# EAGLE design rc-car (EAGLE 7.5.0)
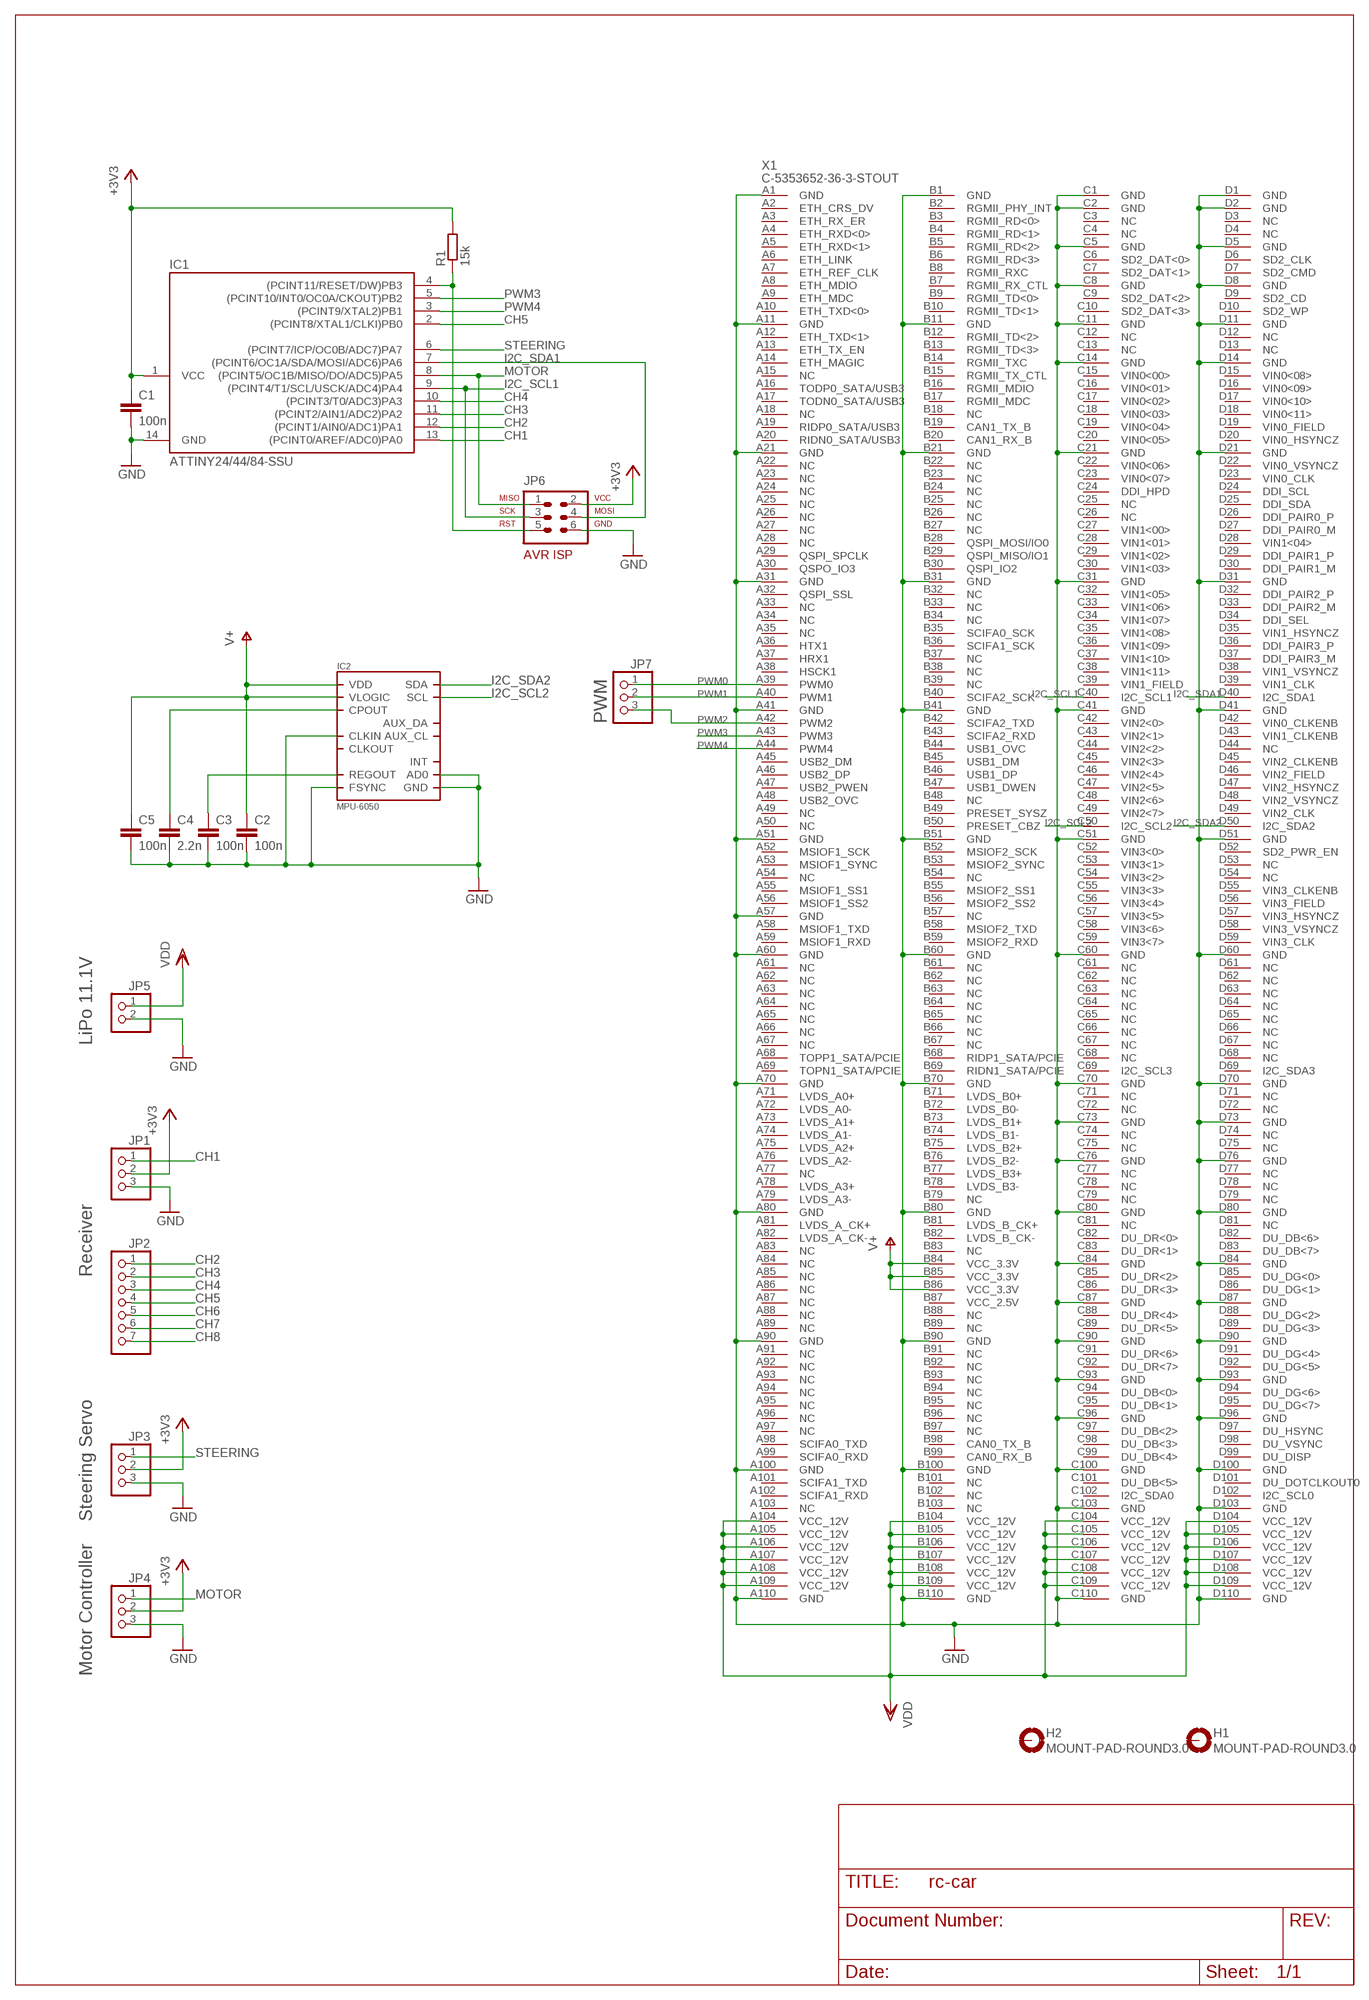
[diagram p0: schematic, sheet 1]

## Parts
C1  100n  C-EUC0805  [C0805]
C2  100n  C-EUC0805  [C0805]
C3  100n  C-EUC0805  [C0805]
C4  2.2n  C-EUC0805  [C0805]
C5  100n  C-EUC0805  [C0805]
H1  MOUNT-PAD-ROUND3.0  [3,0-PAD]
H2  MOUNT-PAD-ROUND3.0  [3,0-PAD]
IC1  ATTINY24/44/84-SSU  [SOIC14]
IC2  MPU-6050  [QFN.24.4X4]
JP1  PINHD-1X3/90  [1X03/90]
JP2  PINHD-1X7/90  [1X07/90]
JP3  PINHD-1X3/90  [1X03/90]
JP4  PINHD-1X3/90  [1X03/90]
JP5  PINHD-1X2  [1X02]
JP6  AVR-ISP-6HORZ  [AVR-ISP-6R]
JP7  PINHD-1X3  [1X03]
R1  15k  R-EU_M0805  [M0805]
X1  C-5353652-36-3-STOUT  [C-5353652-36-3]

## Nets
+3V3: C1.1 IC1.1(VCC) JP1.2 JP3.2 JP4.2 JP6.2 R1.2
CH1: IC1.13((PCINT0/AREF/ADC0)PA0) JP1.1
CH2: IC1.12((PCINT1/AIN0/ADC1)PA1) JP2.1
CH3: IC1.11((PCINT2/AIN1/ADC2)PA2) JP2.2
CH4: IC1.10((PCINT3/T0/ADC3)PA3) JP2.3
CH5: IC1.2((PCINT8/XTAL1/CLKI)PB0) JP2.4
CH6: JP2.5
CH7: JP2.6
CH8: JP2.7
GND: C1.2 C2.2 C3.2 C4.2 C5.2 IC1.14(GND) IC2.1(CLKIN) IC2.9(AD0) IC2.11(FSYNC) IC2.18(GND) JP1.3 JP3.3 JP4.3 JP5.2 JP6.6 X1.A1(GND) X1.A11(GND) X1.A21(GND) X1.A31(GND) X1.A41(GND) X1.A51(GND) X1.A57(GND) X1.A60(GND) X1.A70(GND) X1.A80(GND) X1.A90(GND) X1.A100(GND) X1.A110(GND) X1.B1(GND) X1.B11(GND) X1.B21(GND) X1.B31(GND) X1.B41(GND) X1.B51(GND) X1.B60(GND) X1.B70(GND) X1.B80(GND) X1.B90(GND) X1.B100(GND) X1.B110(GND) X1.C1(GND) X1.C2(GND) X1.C5(GND) X1.C8(GND) X1.C11(GND) X1.C14(GND) X1.C21(GND) X1.C31(GND) X1.C41(GND) X1.C51(GND) X1.C60(GND) X1.C70(GND) X1.C73(GND) X1.C76(GND) X1.C80(GND) X1.C84(GND) X1.C87(GND) X1.C90(GND) X1.C93(GND) X1.C96(GND) X1.C100(GND) X1.C103(GND) X1.C110(GND) X1.D1(GND) X1.D2(GND) X1.D5(GND) X1.D8(GND) X1.D11(GND) X1.D14(GND) X1.D21(GND) X1.D31(GND) X1.D41(GND) X1.D51(GND) X1.D60(GND) X1.D70(GND) X1.D73(GND) X1.D76(GND) X1.D80(GND) X1.D84(GND) X1.D87(GND) X1.D90(GND) X1.D93(GND) X1.D96(GND) X1.D100(GND) X1.D103(GND) X1.D110(GND)
I2C_SCL1: IC1.9((PCINT4/T1/SCL/USCK/ADC4)PA4) JP6.3 X1.C40(I2C_SCL1)
I2C_SCL2: IC2.23(SCL) X1.C50(I2C_SCL2)
I2C_SDA1: IC1.7((PCINT6/OC1A/SDA/MOSI/ADC6)PA6) JP6.4 X1.D40(I2C_SDA1)
I2C_SDA2: IC2.24(SDA) X1.D50(I2C_SDA2)
MOTOR: IC1.8((PCINT5/OC1B/MISO/DO/ADC5)PA5) JP4.1 JP6.1
N$2: IC1.4((PCINT11/RESET/DW)PB3) JP6.5 R1.1
N$4: C3.1 IC2.10(REGOUT)
N$5: C4.1 IC2.20(CPOUT)
PWM0: JP7.1 X1.A39(PWM0)
PWM1: JP7.2 X1.A40(PWM1)
PWM2: JP7.3 X1.A42(PWM2)
PWM3: IC1.5((PCINT10/INT0/OC0A/CKOUT)PB2) X1.A43(PWM3)
PWM4: IC1.3((PCINT9/XTAL2)PB1) X1.A44(PWM4)
STEERING: IC1.6((PCINT7/ICP/OC0B/ADC7)PA7) JP3.1
V+: C2.1 C5.1 IC2.8(VLOGIC) IC2.13(VDD) X1.B84(VCC_3.3V) X1.B85(VCC_3.3V) X1.B86(VCC_3.3V)
VDD: JP5.1 X1.A104(VCC_12V) X1.A105(VCC_12V) X1.A106(VCC_12V) X1.A107(VCC_12V) X1.A108(VCC_12V) X1.A109(VCC_12V) X1.B104(VCC_12V) X1.B105(VCC_12V) X1.B106(VCC_12V) X1.B107(VCC_12V) X1.B108(VCC_12V) X1.B109(VCC_12V) X1.C104(VCC_12V) X1.C105(VCC_12V) X1.C106(VCC_12V) X1.C107(VCC_12V) X1.C108(VCC_12V) X1.C109(VCC_12V) X1.D104(VCC_12V) X1.D105(VCC_12V) X1.D106(VCC_12V) X1.D107(VCC_12V) X1.D108(VCC_12V) X1.D109(VCC_12V)
Unconnected: H1.B3,0(MOUNT) H2.B3,0(MOUNT) IC2.6(AUX_DA) IC2.7(AUX_CL) IC2.12(INT) IC2.22(CLKOUT) X1.A2(ETH_CRS_DV) X1.A3(ETH_RX_ER) X1.A4(ETH_RXD<0>) X1.A5(ETH_RXD<1>) X1.A6(ETH_LINK) X1.A7(ETH_REF_CLK) X1.A8(ETH_MDIO) X1.A9(ETH_MDC) X1.A10(ETH_TXD<0>) X1.A12(ETH_TXD<1>) X1.A13(ETH_TX_EN) X1.A14(ETH_MAGIC) X1.A15(NC) X1.A16(TODP0_SATA/USB3) X1.A17(TODN0_SATA/USB3) X1.A18(NC) X1.A19(RIDP0_SATA/USB3) X1.A20(RIDN0_SATA/USB3) X1.A22(NC) X1.A23(NC) X1.A24(NC) X1.A25(NC) X1.A26(NC) X1.A27(NC) X1.A28(NC) X1.A29(QSPI_SPCLK) X1.A30(QSPO_IO3) X1.A32(QSPI_SSL) X1.A33(NC) X1.A34(NC) X1.A35(NC) X1.A36(HTX1) X1.A37(HRX1) X1.A38(HSCK1) X1.A45(USB2_DM) X1.A46(USB2_DP) X1.A47(USB2_PWEN) X1.A48(USB2_OVC) X1.A49(NC) X1.A50(NC) X1.A52(MSIOF1_SCK) X1.A53(MSIOF1_SYNC) X1.A54(NC) X1.A55(MSIOF1_SS1) X1.A56(MSIOF1_SS2) X1.A58(MSIOF1_TXD) X1.A59(MSIOF1_RXD) X1.A61(NC) X1.A62(NC) X1.A63(NC) X1.A64(NC) X1.A65(NC) X1.A66(NC) X1.A67(NC) X1.A68(TOPP1_SATA/PCIE) X1.A69(TOPN1_SATA/PCIE) X1.A71(LVDS_A0+) X1.A72(LVDS_A0-) X1.A73(LVDS_A1+) X1.A74(LVDS_A1-) X1.A75(LVDS_A2+) X1.A76(LVDS_A2-) X1.A77(NC) X1.A78(LVDS_A3+) X1.A79(LVDS_A3-) X1.A81(LVDS_A_CK+) X1.A82(LVDS_A_CK-) X1.A83(NC) X1.A84(NC) X1.A85(NC) X1.A86(NC) X1.A87(NC) X1.A88(NC) X1.A89(NC) X1.A91(NC) X1.A92(NC) X1.A93(NC) X1.A94(NC) X1.A95(NC) X1.A96(NC) X1.A97(NC) X1.A98(SCIFA0_TXD) X1.A99(SCIFA0_RXD) X1.A101(SCIFA1_TXD) X1.A102(SCIFA1_RXD) X1.A103(NC) X1.B2(RGMII_PHY_INT) X1.B3(RGMII_RD<0>) X1.B4(RGMII_RD<1>) X1.B5(RGMII_RD<2>) X1.B6(RGMII_RD<3>) X1.B7(RGMII_RX_CTL) X1.B8(RGMII_RXC) X1.B9(RGMII_TD<0>) X1.B10(RGMII_TD<1>) X1.B12(RGMII_TD<2>) X1.B13(RGMII_TD<3>) X1.B14(RGMII_TXC) X1.B15(RGMII_TX_CTL) X1.B16(RGMII_MDIO) X1.B17(RGMII_MDC) X1.B18(NC) X1.B19(CAN1_TX_B) X1.B20(CAN1_RX_B) X1.B22(NC) X1.B23(NC) X1.B24(NC) X1.B25(NC) X1.B26(NC) X1.B27(NC) X1.B28(QSPI_MOSI/IO0) X1.B29(QSPI_MISO/IO1) X1.B30(QSPI_IO2) X1.B32(NC) X1.B33(NC) X1.B34(NC) X1.B35(SCIFA0_SCK) X1.B36(SCIFA1_SCK) X1.B37(NC) X1.B38(NC) X1.B39(NC) X1.B40(SCIFA2_SCK) X1.B42(SCIFA2_TXD) X1.B43(SCIFA2_RXD) X1.B44(USB1_OVC) X1.B45(USB1_DM) X1.B46(USB1_DP) X1.B47(USB1_DWEN) X1.B48(NC) X1.B49(PRESET_SYSZ) X1.B50(PRESET_CBZ) X1.B52(MSIOF2_SCK) X1.B53(MSIOF2_SYNC) X1.B54(NC) X1.B55(MSIOF2_SS1) X1.B56(MSIOF2_SS2) X1.B57(NC) X1.B58(MSIOF2_TXD) X1.B59(MSIOF2_RXD) X1.B61(NC) X1.B62(NC) X1.B63(NC) X1.B64(NC) X1.B65(NC) X1.B66(NC) X1.B67(NC) X1.B68(RIDP1_SATA/PCIE) X1.B69(RIDN1_SATA/PCIE) X1.B71(LVDS_B0+) X1.B72(LVDS_B0-) X1.B73(LVDS_B1+) X1.B74(LVDS_B1-) X1.B75(LVDS_B2+) X1.B76(LVDS_B2-) X1.B77(LVDS_B3+) X1.B78(LVDS_B3-) X1.B79(NC) X1.B81(LVDS_B_CK+) X1.B82(LVDS_B_CK-) X1.B83(NC) X1.B87(VCC_2.5V) X1.B88(NC) X1.B89(NC) X1.B91(NC) X1.B92(NC) X1.B93(NC) X1.B94(NC) X1.B95(NC) X1.B96(NC) X1.B97(NC) X1.B98(CAN0_TX_B) X1.B99(CAN0_RX_B) X1.B101(NC) X1.B102(NC) X1.B103(NC) X1.C3(NC) X1.C4(NC) X1.C6(SD2_DAT<0>) X1.C7(SD2_DAT<1>) X1.C9(SD2_DAT<2>) X1.C10(SD2_DAT<3>) X1.C12(NC) X1.C13(NC) X1.C15(VIN0<00>) X1.C16(VIN0<01>) X1.C17(VIN0<02>) X1.C18(VIN0<03>) X1.C19(VIN0<04>) X1.C20(VIN0<05>) X1.C22(VIN0<06>) X1.C23(VIN0<07>) X1.C24(DDI_HPD) X1.C25(NC) X1.C26(NC) X1.C27(VIN1<00>) X1.C28(VIN1<01>) X1.C29(VIN1<02>) X1.C30(VIN1<03>) X1.C32(VIN1<05>) X1.C33(VIN1<06>) X1.C34(VIN1<07>) X1.C35(VIN1<08>) X1.C36(VIN1<09>) X1.C37(VIN1<10>) X1.C38(VIN1<11>) X1.C39(VIN1_FIELD) X1.C42(VIN2<0>) X1.C43(VIN2<1>) X1.C44(VIN2<2>) X1.C45(VIN2<3>) X1.C46(VIN2<4>) X1.C47(VIN2<5>) X1.C48(VIN2<6>) X1.C49(VIN2<7>) X1.C52(VIN3<0>) X1.C53(VIN3<1>) X1.C54(VIN3<2>) X1.C55(VIN3<3>) X1.C56(VIN3<4>) X1.C57(VIN3<5>) X1.C58(VIN3<6>) X1.C59(VIN3<7>) X1.C61(NC) X1.C62(NC) X1.C63(NC) X1.C64(NC) X1.C65(NC) X1.C66(NC) X1.C67(NC) X1.C68(NC) X1.C69(I2C_SCL3) X1.C71(NC) X1.C72(NC) X1.C74(NC) X1.C75(NC) X1.C77(NC) X1.C78(NC) X1.C79(NC) X1.C81(NC) X1.C82(DU_DR<0>) X1.C83(DU_DR<1>) X1.C85(DU_DR<2>) X1.C86(DU_DR<3>) X1.C88(DU_DR<4>) X1.C89(DU_DR<5>) X1.C91(DU_DR<6>) X1.C92(DU_DR<7>) X1.C94(DU_DB<0>) X1.C95(DU_DB<1>) X1.C97(DU_DB<2>) X1.C98(DU_DB<3>) X1.C99(DU_DB<4>) X1.C101(DU_DB<5>) X1.C102(I2C_SDA0) X1.D3(NC) X1.D4(NC) X1.D6(SD2_CLK) X1.D7(SD2_CMD) X1.D9(SD2_CD) X1.D10(SD2_WP) X1.D12(NC) X1.D13(NC) X1.D15(VIN0<08>) X1.D16(VIN0<09>) X1.D17(VIN0<10>) X1.D18(VIN0<11>) X1.D19(VIN0_FIELD) X1.D20(VIN0_HSYNCZ) X1.D22(VIN0_VSYNCZ) X1.D23(VIN0_CLK) X1.D24(DDI_SCL) X1.D25(DDI_SDA) X1.D26(DDI_PAIR0_P) X1.D27(DDI_PAIR0_M) X1.D28(VIN1<04>) X1.D29(DDI_PAIR1_P) X1.D30(DDI_PAIR1_M) X1.D32(DDI_PAIR2_P) X1.D33(DDI_PAIR2_M) X1.D34(DDI_SEL) X1.D35(VIN1_HSYNCZ) X1.D36(DDI_PAIR3_P) X1.D37(DDI_PAIR3_M) X1.D38(VIN1_VSYNCZ) X1.D39(VIN1_CLK) X1.D42(VIN0_CLKENB) X1.D43(VIN1_CLKENB) X1.D44(NC) X1.D45(VIN2_CLKENB) X1.D46(VIN2_FIELD) X1.D47(VIN2_HSYNCZ) X1.D48(VIN2_VSYNCZ) X1.D49(VIN2_CLK) X1.D52(SD2_PWR_EN) X1.D53(NC) X1.D54(NC) X1.D55(VIN3_CLKENB) X1.D56(VIN3_FIELD) X1.D57(VIN3_HSYNCZ) X1.D58(VIN3_VSYNCZ) X1.D59(VIN3_CLK) X1.D61(NC) X1.D62(NC) X1.D63(NC) X1.D64(NC) X1.D65(NC) X1.D66(NC) X1.D67(NC) X1.D68(NC) X1.D69(I2C_SDA3) X1.D71(NC) X1.D72(NC) X1.D74(NC) X1.D75(NC) X1.D77(NC) X1.D78(NC) X1.D79(NC) X1.D81(NC) X1.D82(DU_DB<6>) X1.D83(DU_DB<7>) X1.D85(DU_DG<0>) X1.D86(DU_DG<1>) X1.D88(DU_DG<2>) X1.D89(DU_DG<3>) X1.D91(DU_DG<4>) X1.D92(DU_DG<5>) X1.D94(DU_DG<6>) X1.D95(DU_DG<7>) X1.D97(DU_HSYNC) X1.D98(DU_VSYNC) X1.D99(DU_DISP) X1.D101(DU_DOTCLKOUT0) X1.D102(I2C_SCL0)

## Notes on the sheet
- PWM
- LiPo 11.1V
- Receiver
- Steering Servo
- Motor Controller

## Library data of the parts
C1-C5 = rcl:C-EU: CAPACITOR, European symbol
H1 H2 = holes:MOUNT-PAD-ROUND: MOUNTING PAD, round
IC1 = attiny24_44_84:ATTINY24/44/84
IC2 = MPU6050:MPU-6050
JP1 JP3 JP4 JP7 = pinhead:PINHD-1X3: PIN HEADER
JP2 = pinhead:PINHD-1X7: PIN HEADER
JP5 = pinhead:PINHD-1X2: PIN HEADER
JP6 = avr-7:AVR-ISP-6: AVR ISP-6 Serial Programming Header
R1 = rcl:R-EU_: RESISTOR, European symbol
X1 = con-tyco:C-5353652-36-3-STOUT

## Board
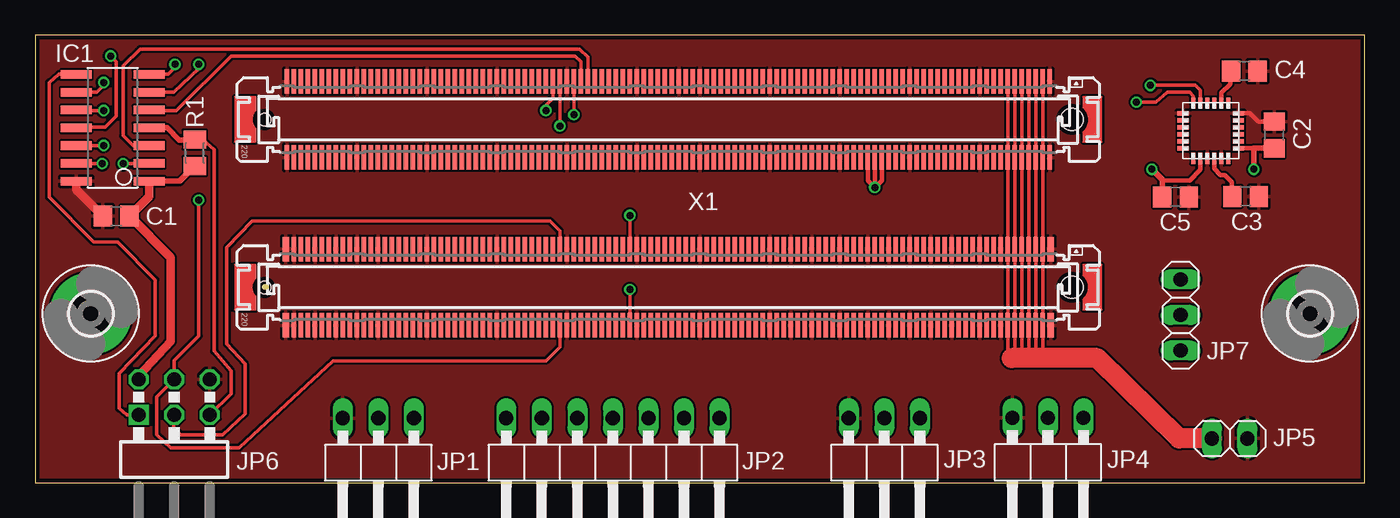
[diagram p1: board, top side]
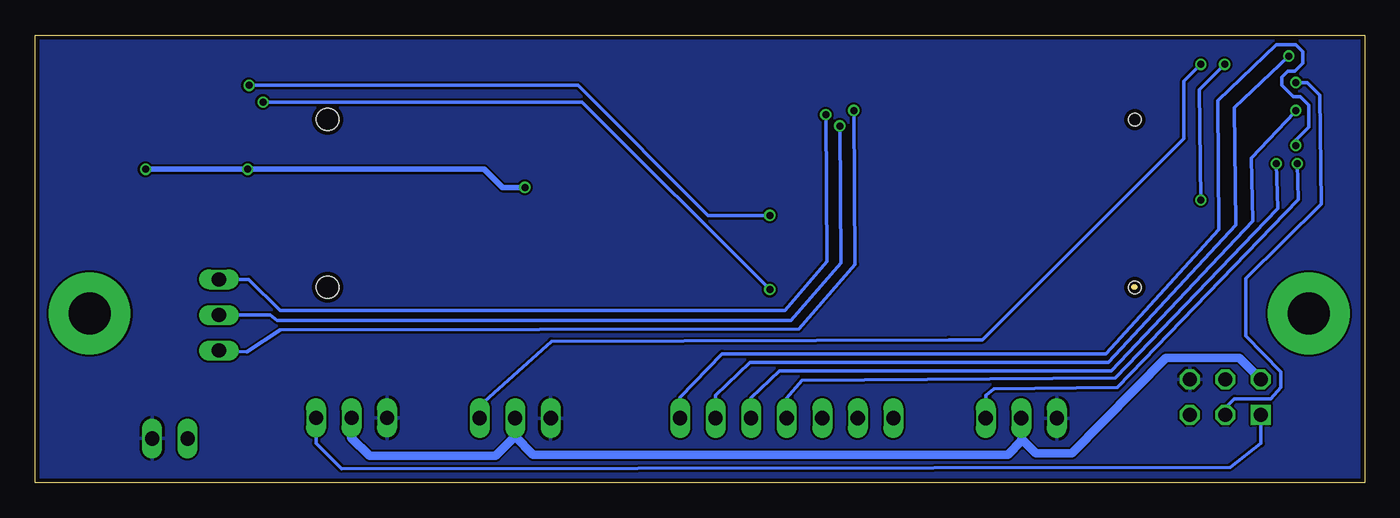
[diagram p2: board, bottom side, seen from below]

Size 95 x 32 mm. Coordinates in mm from the lower left corner, seen from the top.
Outline: 16.4,14 16.5,14
Outline: 0,0 95,0 95,32 0,32 0,0
Copper layers (1*16): Top 0.035mm / dielectric 1.5mm / Bottom 0.035mm
Design rules "PCB-POOL Standard": minimum track width 0.15mm, minimum drill 0.3mm, track to track 0.15mm, track to pad 0.15mm, pad to pad 0.15mm, via to via 0.15mm, smd to smd 0.15mm, copper to edge 0.3mm, drill to drill 0.2mm, minimum pad ring 0.2mm, minimum via ring 0.15mm, stop-mask expansion 0.075mm, vias tented up to drill 0mil, thermal gap 0.2mm

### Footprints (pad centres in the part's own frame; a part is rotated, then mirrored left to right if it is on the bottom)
C0805 = smd 1.3 x 1.5: 1 -0.95,0; 2 0.95,0
3,0-PAD = drill 3 pad 5.842: B3,0 0,0
SOIC14 = smd 0.61 x 2.21: 1 -3.81,-2.603; 2 -2.54,-2.603; 3 -1.27,-2.603; 4 0,-2.603; 5 1.27,-2.603; 6 2.54,-2.603; 7 3.81,-2.603; 8 3.81,2.603; 9 2.54,2.603; 10 1.27,2.603; 11 0,2.603; 12 -1.27,2.603; 13 -2.54,2.603; 14 -3.81,2.603
QFN.24.4X4 = smd 0.8 x 0.3: 1 -1.975,1.25; 2 -1.975,0.75; 3 -1.975,0.25; 4 -1.975,-0.25; 5 -1.975,-0.75; 6 -1.975,-1.25; 13 1.975,-1.25; 14 1.975,-0.75; 15 1.975,-0.25; 16 1.975,0.25; 17 1.975,0.75; 18 1.975,1.25 | smd 0.3 x 0.8: 7 -1.25,-1.975; 8 -0.75,-1.975; 9 -0.25,-1.975; 10 0.25,-1.975; 11 0.75,-1.975; 12 1.25,-1.975; 19 1.25,1.975; 20 0.75,1.975; 21 0.25,1.975; 22 -0.25,1.975; 23 -0.75,1.975; 24 -1.25,1.975
1X03/90 = drill 1.016 long: 1 -2.54,-3.81; 2 0,-3.81; 3 2.54,-3.81
1X07/90 = drill 1.016 long: 1 -7.62,-3.81; 2 -5.08,-3.81; 3 -2.54,-3.81; 4 0,-3.81; 5 2.54,-3.81; 6 5.08,-3.81; 7 7.62,-3.81
1X02 = drill 1.016 long: 1 -1.27,0; 2 1.27,0
AVR-ISP-6R = drill 1.016 square: 1 -2.54,-1.27 | drill 1.016 octagon: 2 -2.54,1.27; 3 0,-1.27; 4 0,1.27; 5 2.54,-1.27; 6 2.54,1.27
1X03 = drill 1.016 long: 1 -2.54,0; 2 0,0; 3 2.54,0
M0805 = smd 1.3 x 1.6: 1 -0.95,0; 2 0.95,0
C-5353652-36-3 = smd 0.3 x 1.75: A1 -27.25,8.705; A2 -26.75,8.705; A3 -26.25,8.705; A4 -25.75,8.705; A5 -25.25,8.705; A6 -24.75,8.705; A7 -24.25,8.705; A8 -23.75,8.705; A9 -23.25,8.705; A10 -22.75,8.705; A11 -22.25,8.705; A12 -21.75,8.705; A13 -21.25,8.705; A14 -20.75,8.705; A15 -20.25,8.705; A16 -19.75,8.705; A17 -19.25,8.705; A18 -18.75,8.705; A19 -18.25,8.705; A20 -17.75,8.705; A21 -17.25,8.705; A22 -16.75,8.705; A23 -16.25,8.705; A24 -15.75,8.705; A25 -15.25,8.705; A26 -14.75,8.705; A27 -14.25,8.705; A28 -13.75,8.705; A29 -13.25,8.705; A30 -12.75,8.705; A31 -12.25,8.705; A32 -11.75,8.705; A33 -11.25,8.705; A34 -10.75,8.705; A35 -10.25,8.705; A36 -9.75,8.705; A37 -9.25,8.705; A38 -8.75,8.705; A39 -8.25,8.705; A40 -7.75,8.705; A41 -7.25,8.705; A42 -6.75,8.705; A43 -6.25,8.705; A44 -5.75,8.705; A45 -5.25,8.705; A46 -4.75,8.705; A47 -4.25,8.705; A48 -3.75,8.705; A49 -3.25,8.705; A50 -2.75,8.705; A51 -2.25,8.705; A52 -1.75,8.705; A53 -1.25,8.705; A54 -0.75,8.705; A55 -0.25,8.705; A56 0.25,8.705; A57 0.75,8.705; A58 1.25,8.705; A59 1.75,8.705; A60 2.25,8.705; A61 2.75,8.705; A62 3.25,8.705; A63 3.75,8.705; A64 4.25,8.705; A65 4.75,8.705; A66 5.25,8.705; A67 5.75,8.705; A68 6.25,8.705; A69 6.75,8.705; A70 7.25,8.705; A71 7.75,8.705; A72 8.25,8.705; A73 8.75,8.705; A74 9.25,8.705; A75 9.75,8.705; A76 10.25,8.705; A77 10.75,8.705; A78 11.25,8.705; A79 11.75,8.705; A80 12.25,8.705; A81 12.75,8.705; A82 13.25,8.705; A83 13.75,8.705; A84 14.25,8.705; A85 14.75,8.705; A86 15.25,8.705; A87 15.75,8.705; A88 16.25,8.705; A89 16.75,8.705; A90 17.25,8.705; A91 17.75,8.705; A92 18.25,8.705; A93 18.75,8.705; A94 19.25,8.705; A95 19.75,8.705; A96 20.25,8.705; A97 20.75,8.705; A98 21.25,8.705; A99 21.75,8.705; A100 22.25,8.705; A101 22.75,8.705; A102 23.25,8.705; A103 23.75,8.705; A104 24.25,8.705; A105 24.75,8.705; A106 25.25,8.705; A107 25.75,8.705; A108 26.25,8.705; A109 26.75,8.705; A110 27.25,8.705; B1 -27.25,3.275; B2 -26.75,3.275; B3 -26.25,3.275; B4 -25.75,3.275; B5 -25.25,3.275; B6 -24.75,3.275; B7 -24.25,3.275; B8 -23.75,3.275; B9 -23.25,3.275; B10 -22.75,3.275; B11 -22.25,3.275; B12 -21.75,3.275; B13 -21.25,3.275; B14 -20.75,3.275; B15 -20.25,3.275; B16 -19.75,3.275; B17 -19.25,3.275; B18 -18.75,3.275; B19 -18.25,3.275; B20 -17.75,3.275; B21 -17.25,3.275; B22 -16.75,3.275; B23 -16.25,3.275; B24 -15.75,3.275; B25 -15.25,3.275; B26 -14.75,3.275; B27 -14.25,3.275; B28 -13.75,3.275; B29 -13.25,3.275; B30 -12.75,3.275; B31 -12.25,3.275; B32 -11.75,3.275; B33 -11.25,3.275; B34 -10.75,3.275; B35 -10.25,3.275; B36 -9.75,3.275; B37 -9.25,3.275; B38 -8.75,3.275; B39 -8.25,3.275; B40 -7.75,3.275; B41 -7.25,3.275; B42 -6.75,3.275; B43 -6.25,3.275; B44 -5.75,3.275; B45 -5.25,3.275; B46 -4.75,3.275; B47 -4.25,3.275; B48 -3.75,3.275; B49 -3.25,3.275; B50 -2.75,3.275; B51 -2.25,3.275; B52 -1.75,3.275; B53 -1.25,3.275; B54 -0.75,3.275; B55 -0.25,3.275; B56 0.25,3.275; B57 0.75,3.275; B58 1.25,3.275; B59 1.75,3.275; B60 2.25,3.275; B61 2.75,3.275; B62 3.25,3.275; B63 3.75,3.275; B64 4.25,3.275; B65 4.75,3.275; B66 5.25,3.275; B67 5.75,3.275; B68 6.25,3.275; B69 6.75,3.275; B70 7.25,3.275; B71 7.75,3.275; B72 8.25,3.275; B73 8.75,3.275; B74 9.25,3.275; B75 9.75,3.275; B76 10.25,3.275; B77 10.75,3.275; B78 11.25,3.275; B79 11.75,3.275; B80 12.25,3.275; B81 12.75,3.275; B82 13.25,3.275; B83 13.75,3.275; B84 14.25,3.275; B85 14.75,3.275; B86 15.25,3.275; B87 15.75,3.275; B88 16.25,3.275; B89 16.75,3.275; B90 17.25,3.275; B91 17.75,3.275; B92 18.25,3.275; B93 18.75,3.275; B94 19.25,3.275; B95 19.75,3.275; B96 20.25,3.275; B97 20.75,3.275; B98 21.25,3.275; B99 21.75,3.275; B100 22.25,3.275; B101 22.75,3.275; B102 23.25,3.275; B103 23.75,3.275; B104 24.25,3.275; B105 24.75,3.275; B106 25.25,3.275; B107 25.75,3.275; B108 26.25,3.275; B109 26.75,3.275; B110 27.25,3.275; C2 -26.75,-3.275; C3 -26.25,-3.275; C4 -25.75,-3.275; C5 -25.25,-3.275; C6 -24.75,-3.275; C7 -24.25,-3.275; C8 -23.75,-3.275; C9 -23.25,-3.275; C10 -22.75,-3.275; C11 -22.25,-3.275; C12 -21.75,-3.275; C13 -21.25,-3.275; C14 -20.75,-3.275; C15 -20.25,-3.275; C16 -19.75,-3.275; C17 -19.25,-3.275; C18 -18.75,-3.275; C19 -18.25,-3.275; C20 -17.75,-3.275; C21 -17.25,-3.275; C22 -16.75,-3.275; C23 -16.25,-3.275; C24 -15.75,-3.275; C25 -15.25,-3.275; C26 -14.75,-3.275; C27 -14.25,-3.275; C28 -13.75,-3.275; C29 -13.25,-3.275; C30 -12.75,-3.275; C31 -12.25,-3.275; C32 -11.75,-3.275; C33 -11.25,-3.275; C34 -10.75,-3.275; C35 -10.25,-3.275; C36 -9.75,-3.275; C37 -9.25,-3.275; C38 -8.75,-3.275; C39 -8.25,-3.275; C40 -7.75,-3.275; C41 -7.25,-3.275; C42 -6.75,-3.275; C43 -6.25,-3.275; C44 -5.75,-3.275; C45 -5.25,-3.275; C46 -4.75,-3.275; C47 -4.25,-3.275; C48 -3.75,-3.275; C49 -3.25,-3.275; C50 -2.75,-3.275; C51 -2.25,-3.275; C52 -1.75,-3.275; C53 -1.25,-3.275; C54 -0.75,-3.275; C55 -0.25,-3.275; C56 0.25,-3.275; C57 0.75,-3.275; C58 1.25,-3.275; C59 1.75,-3.275; C60 2.25,-3.275; C61 2.75,-3.275; C62 3.25,-3.275; C63 3.75,-3.275; C64 4.25,-3.275; C65 4.75,-3.275; C66 5.25,-3.275; C67 5.75,-3.275; C68 6.25,-3.275; C69 6.75,-3.275; C70 7.25,-3.275; C71 7.75,-3.275; C72 8.25,-3.275; C73 8.75,-3.275; C74 9.25,-3.275; C75 9.75,-3.275; C76 10.25,-3.275; C77 10.75,-3.275; C78 11.25,-3.275; C79 11.75,-3.275; C80 12.25,-3.275; C81 12.75,-3.275; C82 13.25,-3.275; C83 13.75,-3.275; C84 14.25,-3.275; C85 14.75,-3.275; C86 15.25,-3.275; C87 15.75,-3.275; C88 16.25,-3.275; C89 16.75,-3.275; C90 17.25,-3.275; C91 17.75,-3.275; C92 18.25,-3.275; C93 18.75,-3.275; C94 19.25,-3.275; C95 19.75,-3.275; C96 20.25,-3.275; C97 20.75,-3.275; C98 21.25,-3.275; C99 21.75,-3.275; C100 22.25,-3.275; C101 22.75,-3.275; C102 23.25,-3.275; C103 23.75,-3.275; C104 24.25,-3.275; C105 24.75,-3.275; C106 25.25,-3.275; C107 25.75,-3.275; C108 26.25,-3.275; C109 26.75,-3.275; D2 -26.75,-8.725; D3 -26.25,-8.725; D4 -25.75,-8.725; D5 -25.25,-8.725; D6 -24.75,-8.725; D7 -24.25,-8.725; D8 -23.75,-8.725; D9 -23.25,-8.725; D10 -22.75,-8.725; D11 -22.25,-8.725; D12 -21.75,-8.725; D13 -21.25,-8.725; D14 -20.75,-8.725; D15 -20.25,-8.725; D16 -19.75,-8.725; D17 -19.25,-8.725; D18 -18.75,-8.725; D19 -18.25,-8.725; D20 -17.75,-8.725; D21 -17.25,-8.725; D22 -16.75,-8.725; D23 -16.25,-8.725; D24 -15.75,-8.725; D25 -15.25,-8.725; D26 -14.75,-8.725; D27 -14.25,-8.725; D28 -13.75,-8.725; D29 -13.25,-8.725; D30 -12.75,-8.725; D31 -12.25,-8.725; D32 -11.75,-8.725; D33 -11.25,-8.725; D34 -10.75,-8.725; D35 -10.25,-8.725; D36 -9.75,-8.725; D37 -9.25,-8.725; D38 -8.75,-8.725; D39 -8.25,-8.725; D40 -7.75,-8.725; D41 -7.25,-8.725; D42 -6.75,-8.725; D43 -6.25,-8.725; D44 -5.75,-8.725; D45 -5.25,-8.725; D46 -4.75,-8.725; D47 -4.25,-8.725; D48 -3.75,-8.725; D49 -3.25,-8.725; D50 -2.75,-8.725; D51 -2.25,-8.725; D52 -1.75,-8.725; D53 -1.25,-8.725; D54 -0.75,-8.725; D55 -0.25,-8.725; D56 0.25,-8.725; D57 0.75,-8.725; D58 1.25,-8.725; D59 1.75,-8.725; D60 2.25,-8.725; D61 2.75,-8.725; D62 3.25,-8.725; D63 3.75,-8.725; D64 4.25,-8.725; D65 4.75,-8.725; D66 5.25,-8.725; D67 5.75,-8.725; D68 6.25,-8.725; D69 6.75,-8.725; D70 7.25,-8.725; D71 7.75,-8.725; D72 8.25,-8.725; D73 8.75,-8.725; D74 9.25,-8.725; D75 9.75,-8.725; D76 10.25,-8.725; D77 10.75,-8.725; D78 11.25,-8.725; D79 11.75,-8.725; D80 12.25,-8.725; D81 12.75,-8.725; D82 13.25,-8.725; D83 13.75,-8.725; D84 14.25,-8.725; D85 14.75,-8.725; D86 15.25,-8.725; D87 15.75,-8.725; D88 16.25,-8.725; D89 16.75,-8.725; D90 17.25,-8.725; D91 17.75,-8.725; D92 18.25,-8.725; D93 18.75,-8.725; D94 19.25,-8.725; D95 19.75,-8.725; D96 20.25,-8.725; D97 20.75,-8.725; D98 21.25,-8.725; D99 21.75,-8.725; D100 22.25,-8.725; D101 22.75,-8.725; D102 23.25,-8.725; D103 23.75,-8.725; D104 24.25,-8.725; D105 24.75,-8.725; D106 25.25,-8.725; D107 25.75,-8.725; D108 26.25,-8.725; D109 26.75,-8.725 | smd 0.45 x 1.75: C1 -27.325,-3.275; C110 27.325,-3.275; D1 -27.325,-8.725; D110 27.325,-8.725 | hole 0.9: -28.85,-6; -28.85,6; -28.85,-6 | hole 1.6: 28.85,-6; 28.85,6; 28.85,-6

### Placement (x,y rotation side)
C1  5.8,19.05 180 top
C2  88.55,24.85 90 top
C3  86.5,20.45 0 top
C4  86.41,29.42 0 top
C5  81.49,20.42 0 top
H1  3.99,12.08 0 top
H2  91.1,12.08 0 top
IC1  5.55,25.36 90 top
IC2  84.01,25.15 0 top
JP1  24.53,0.79 180 top
JP2  41.29,0.79 180 top
JP3  60.69,0.79 180 top
JP4  72.38,0.81 180 top
JP5  85.36,3.15 0 top
JP6  9.95,6.1 0 top
JP7  81.85,11.98 90 top
R1  11.42,23.57 270 top
X1  45.25,19.96 0 top

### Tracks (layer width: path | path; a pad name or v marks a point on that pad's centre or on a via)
+3V3
  Top 0.406: IC1.1 10.35,21.55 R1.2
  Top 0.61: IC1.1 8.15,20.45 C1.1 9.7,16.1 9.7,10.1 7.41,7.61 JP6.2
  Bottom 0.61: JP4.2 72.4,4.6 72.4,3.2 71.1,1.9 62.1,1.9 60.69,3.31 JP3.2 60.7,3.3 59.4,2 25.5,2 24.53,2.97 JP1.2 24.5,4.57 24.5,3.1 23.5,2.1 20.9,2.1 14.2,8.9 8.94,8.9 JP6.2 7.41,7.39 7.4,7.4
CH1  (via drill 0.5)
  Top 0.254: v4.8,22.8 2.93,22.8 IC1.13
  Bottom 0.254: JP1.1 27.07,6.23 26.5,6.7 17.67,6.8 4.75,20.22 4.82,22.82 v4.8,22.8
CH2  (via drill 0.5)
  Top 0.254: IC1.12 2.94,24.1 v4.9,24.1
  Bottom 0.254: JP2.1 48.91,6.09 45.9,9.2 18.5,9.2 10.4,18.1 10.5,27.3 6.3,31.3 4.9,31.3 4.4,30.8 4.4,30 5,29.4 5.5,29.4 5.9,29 5.9,28.4 5.1,27.6 4.6,27.6 4,27 4,25.4 4.9,24.5 v4.9,24.1
CH3  (via drill 0.5)
  Top 0.254: IC1.11 2.99,25.4 5,25.4 5.8,26.2 5.8,30.1 v5.4,30.5
  Bottom 0.254: JP2.2 46.37,6.23 43.9,8.6 18.3,8.6 9.2,18.4 9.3,26.8 v5.4,30.5
CH4  (via drill 0.5)
  Top 0.254: v4.9,26.6 2.88,26.6 IC1.10
  Bottom 0.254: JP2.3 43.83,6.07 41.8,8 18.1,8 8,18.7 8.1,23.2 5,26.5 | 5,26.5 5.1,26.5 | 5,26.5 v4.9,26.6
CH5  (via drill 0.5)
  Top 0.254: v6.3,22.8 8.13,22.8 IC1.2
  Bottom 0.254: JP2.4 41.29,6.01 40.2,7.3 17.8,7.5 6.2,19.6 v6.3,22.8
GND
  Top 0.305: IC2.18 86.8,26.4 87.4,25.8 C2.2
  Top 0.61: IC1.14 2.95,20.95 C1.2
  pour Top: 0.2,31.8 94.8,31.8 94.8,0.2 0.2,0.2 0.2,31.7
  pour Bottom: 0.3,31.7 94.7,31.7 94.7,0.4 0.3,0.4 0.3,31.6
I2C_SCL1  (via drill 0.5)
  Top 0.254: X1.C40 37.5,18 36.8,18.7 15.5,18.7 13.7,16.8 13.7,9.9 15,8.5 15,4.9 13.4,3.4 10.4,3.4 9.9,3.9 9.9,4.78 JP6.3 | v4.9,28.6 4.9,28.4 4.4,27.9 IC1.9
  Bottom 0.254: JP6.3 9.95,5.35 9.3,6 6.7,6 6,6.8 6,7.9 8.5,10.5 8.5,14.6 3.1,19.9 3.2,27.7 4.1,28.6 v4.9,28.6
I2C_SCL2  (via drill 0.5)
  Top 0.254: IC2.23 83.26,28.04 82.9,28.4 v79.7,28.4 | v42.5,19.1 X1.C50
  Bottom 0.254: v79.7,28.4 56.2,28.4 46.9,19.1 v42.5,19.1
I2C_SDA1  (via drill 0.5)
  Top 0.254: X1.D40 37.5,9.7 36.5,8.7 21.3,8.7 14.6,2.5 9.7,2.5 8.7,3.4 8.7,6.12 JP6.4 9.95,8.75 11.7,10.5 v11.7,20.2 | v10,29.9 9.9,29.6 9.5,29.2 8.18,29.2 IC1.7
  Bottom 0.254: v11.7,20.2 11.8,28.1 v10,29.9
I2C_SDA2  (via drill 0.5)
  Top 0.254: IC2.24 82.78,27.62 82.5,27.9 80.9,27.9 80.1,27.2 v78.7,27.2 | v42.5,13.8 X1.D50
  Bottom 0.254: v78.7,27.2 55.9,27.2 v42.5,13.8
MOTOR
  Top 0.254: JP6.1 6.57,4.83 6,5.3 6,7.8 8.6,10.5 8.6,14.5 5.9,17.2 4.2,17.2 1,20.4 1,28.6 1.7,29.2 2.92,29.2 IC1.8
  Bottom 0.254: JP4.1 74.92,2.82 73.1,1 9.6,1.1 7.4,2.8 JP6.1
N$2
  Top 0.254: 11.4,24.5 12,24.5 12.8,23.8 12.8,9.4 14,8 14,6.34 JP6.5
  Top 0.406: IC1.4 9.44,25.36 10.3,24.5 11.4,24.5 R1.1
N$4
  Top 0.305: IC2.10 84.26,22.44 84.7,22 85,22 85.5,21.5 85.5,20.5
  Top 0.406: 85.5,20.5 C3.1
N$5
  Top 0.305: IC2.20 84.76,27.86 85.4,28.5 85.4,29.36
  Top 0.406: 85.4,29.36 C4.1
PWM0  (via drill 0.5)
  Top 0.254: v36.5,26.6 36.5,27 37,27.5 X1.A39
  Bottom 0.254: JP7.1 79.86,9.34 77.5,10.9 40.4,11 36.4,15.6 v36.5,26.6
PWM1  (via drill 0.5)
  Top 0.254: v37.5,25.5 X1.A40
  Bottom 0.254: JP7.2 78.18,11.98 77.7,11.6 41,11.6 37.4,15.7 v37.5,25.5
PWM2  (via drill 0.5)
  Top 0.254: v38.5,26.3 X1.A42
  Bottom 0.254: JP7.3 79.72,14.52 77.5,12.3 41.4,12.3 38.4,15.8 v38.5,26.3
PWM3
  Top 0.254: X1.A43 39,30.1 38.6,30.5 14,30.5 10.1,26.6 8.18,26.6 IC1.5
PWM4
  Top 0.254: X1.A44 39.5,30.4 38.9,31 7.5,31 6.3,29.8 6.3,24.8 7,24.1 IC1.3
STEERING  (via drill 0.5)
  Top 0.254: v11.7,29.9 11.7,29.6 9.9,27.9 IC1.6
  Bottom 0.254: JP3.1 63.23,5.47 58.1,10.1 29.7,10.2 27.3,10.2 12.9,24.6 12.9,28.7 v11.7,29.9
V+  (via drill 0.5)
  Top 0.305: IC2.13 87.1,23.9 | v60,21.1 X1.B85 | X1.B86 60.5,21.6 v60,21.1 | X1.B84 59.5,21.6 v60,21.1 | IC2.8 83.26,22.36 82.5,21.6 80.58,21.6 80.54,21.66
  Top 0.406: C2.1 87.1,23.9 v87.1,22.4 | C5.1 80.54,21.66 v79.8,22.4
  Bottom 0.406: v87.1,22.4 v79.8,22.4 62.9,22.4 61.6,21.1 v60,21.1
VDD
  Top 0.254: X1.A108 X1.B108 X1.C108 X1.D108 71.5,8.9 | X1.A109 X1.B109 X1.C109 X1.D109 72,8.9 71.5,8.9 | X1.A107 X1.B107 X1.C107 X1.D107 71,8.9 | X1.A106 X1.B106 X1.C106 X1.D106 70.5,8.9 | X1.A105 X1.B105 X1.C105 X1.D105 70,8.9 | X1.A104 X1.B104 X1.C104 X1.D104 69.5,8.9 69.8,8.9 70,8.9 | 71.5,8.9 71,8.9 | 71,8.9 70.5,8.9 | 70.5,8.9 70,8.9
  Top 1.422: JP5.1 81.75,3.15 75.9,8.9 69.8,8.9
